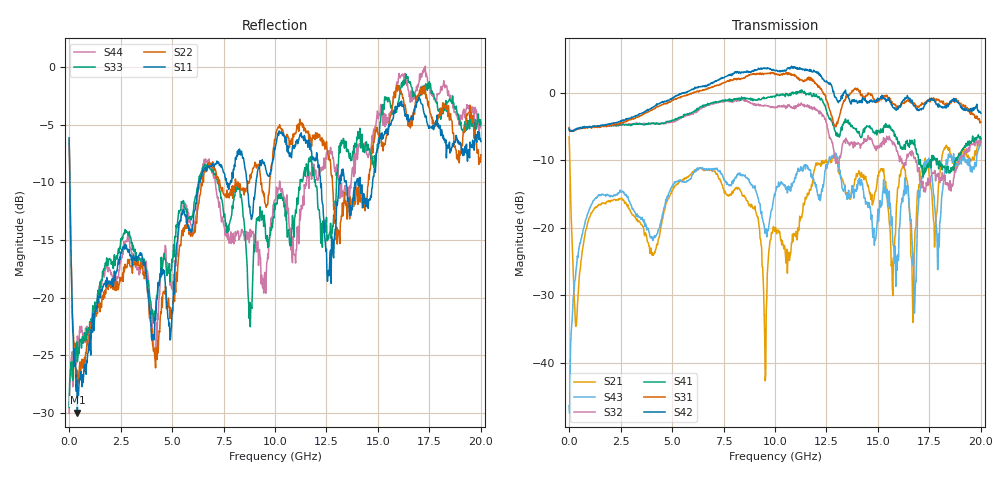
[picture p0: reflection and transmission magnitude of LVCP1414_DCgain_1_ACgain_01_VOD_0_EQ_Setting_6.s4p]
!Agilent Technologies,N5230A,MY46400459,A.07.50.48
!Agilent N5230A: A.07.50.48
!Date: Tuesday, April 17, 2012 18:46:55
!Correction: S11(Full 4 Port(1,2,3,4))
!S12(Full 4 Port(1,2,3,4))
!S13(Full 4 Port(1,2,3,4))
!S14(Full 4 Port(1,2,3,4))
!S21(Full 4 Port(1,2,3,4))
!S22(Full 4 Port(1,2,3,4))
!S23(Full 4 Port(1,2,3,4))
!S24(Full 4 Port(1,2,3,4))
!S31(Full 4 Port(1,2,3,4))
!S32(Full 4 Port(1,2,3,4))
!S33(Full 4 Port(1,2,3,4))
!S34(Full 4 Port(1,2,3,4))
!S41(Full 4 Port(1,2,3,4))
!S42(Full 4 Port(1,2,3,4))
!S43(Full 4 Port(1,2,3,4))
!S44(Full 4 Port(1,2,3,4))
!S4P File: Measurements: <S11,S12,S13,S14>,
!<S21,S22,S23,S24>,
!<S31,S32,S33,S34>,
!<S41,S42,S43,S44>:
# Hz S  dB  R 50
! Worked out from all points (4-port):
!   801 points, 300 kHz to 20 GHz, reference 50 ohm
!   strongest paths, dB at 300 kHz, 5 GHz, 10 GHz, 15 GHz, 20 GHz:
!     S42: -5.3, -0.8, 3.3, -0.8, -3.0
!     S31: -5.1, -1.1, 2.7, -1.3, -4.3
!     S41: -5.2, -4.0, -0.6, -5.5, -6.9
!     S32: -5.2, -4.3, -2.2, -8.2, -7.3
!     S43: -46.4, -13.9, -15.2, -17.2, -7.1
!     S21: -6.5, -14.4, -20.5, -12.2, -7.2
!   lowest |S11| = -29.9 dB at 400.3 MHz (marker M1), VSWR 1.07, Z = 53 + j1.3 ohm
!   |S11| at or under -10 dB: 37.36 MHz to 6.306 GHz (6.269 GHz wide, 198 % of centre); 12.21 GHz to 13.11 GHz (899.7 MHz wide, 7.1 % of centre); 14.14 GHz to 14.74 GHz (602.8 MHz wide, 4.17 % of centre)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
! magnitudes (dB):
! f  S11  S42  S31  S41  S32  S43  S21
! 300 kHz  -6.1  -5.3  -5.1  -5.2  -5.2  -46.4  -6.5
! 400.3 MHz  -29.9  -5.2  -5.3  -5.3  -5.3  -24.2  -31.7
! 9.975 GHz  -7.0  3.4  2.8  -0.6  -2.2  -15.0  -20.0
! 12.73 GHz  -18.8  1.3  -3.2  -4.1  -6.9  -9.8  -10.0
! 16.8 GHz  -3.5  -1.9  -1.7  -7.9  -9.5  -30.0  -20.5
! 17.38 GHz  -4.8  -1.4  -1.1  -10.9  -13.7  -10.0  -10.5
! 20 GHz  -6.5  -3.0  -4.3  -6.9  -7.3  -7.1  -7.2
